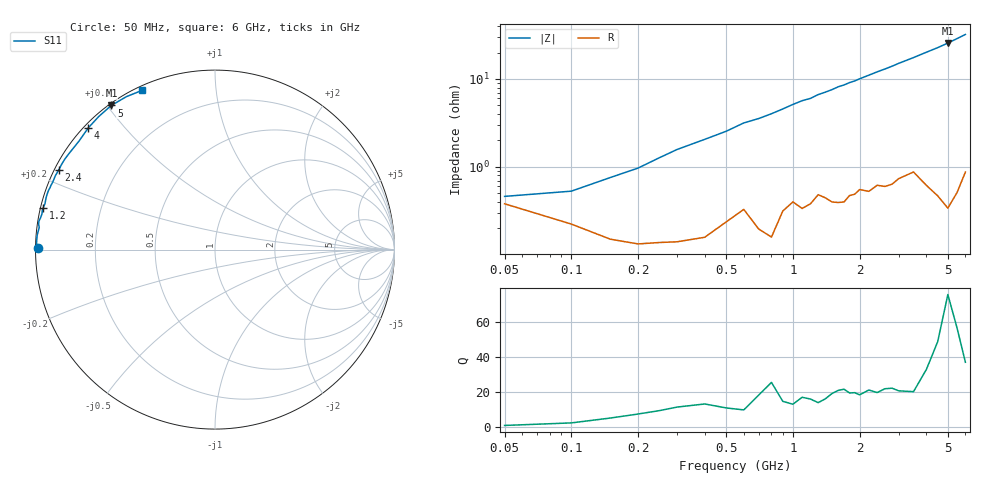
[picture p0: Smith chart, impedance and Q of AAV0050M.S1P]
! Infineon Technologies  Discrete & RF Semiconductors
! BBY66-02W
! Si Tuning Diode in SCD-80
! VR =
! S-Parameters:  June  2000
# GHz  S  MA  R  50
!  f  S11
! GHz  MAG  ANG
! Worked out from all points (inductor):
!   34 points, 50 MHz to 6 GHz, reference 50 ohm
!   read as one part to ground: L = 787 pH near 150 MHz
!   highest Q = 56.5 at 5 GHz (marker M1), where L = 816 pH
!   S11 on the Smith chart (normalised r, x): 50 MHz: 0.01, +0.01; 1.2 GHz: 0.01, +0.12; 2.4 GHz: 0.01, +0.24; 4 GHz: 0.01, +0.40; 5 GHz: 0.01, +0.51; 6 GHz: 0.02, +0.64
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0.05  0.9849 179.4
0.1  0.9911 178.9
0.2  0.9947 177.8
0.3  0.9944 176.4
0.4  0.9937 175.3
0.5  0.9906 174.2
0.6  0.987 172.8
0.7  0.9922 171.9
0.8  0.9937 170.8
1  0.9843 168.3
1.1  0.9868 167.1
1.2  0.9851 166.3
1.3  0.9812 164.9
1.5  0.9845 162.8
1.6  0.9848 161.5
1.9  0.9813 158.5
2  0.979 157.3
2.2  0.9801 155.1
2.4  0.9769 152.9
2.6  0.9778 150.9
2.8  0.9767 148.8
3  0.9734 146.5
3.5  0.9693 141.4
4  0.979 136.1
4.5  0.9846 131.1
5  0.9893 125.7
5.5  0.9848 120.1
6  0.9756 114.6
